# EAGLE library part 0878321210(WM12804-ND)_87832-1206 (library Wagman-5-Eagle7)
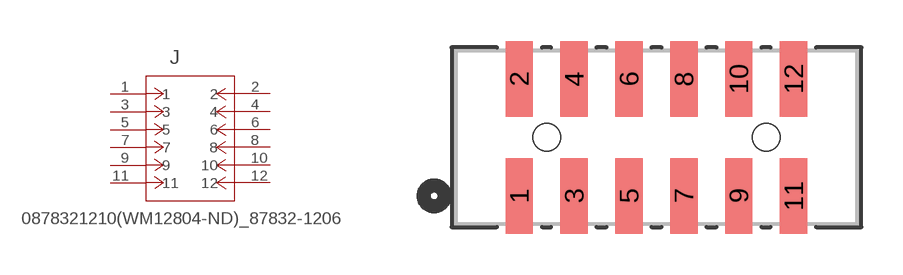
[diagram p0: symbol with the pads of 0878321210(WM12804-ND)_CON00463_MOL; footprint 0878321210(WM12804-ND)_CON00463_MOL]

Designator prefix J

## 0878321210(WM12804-ND)_87832-1206 (BUILT_BY: EMA_Don; COPYRIGHT: Copyright (C) 2016 Accelerated Designs. All rights reserved; MANUFACTURER_PART_NUMBER: 87832-1206; SOURCELIBRARY: Molex_2018-12-15; VENDOR: Molex Connector Corporation)  [0878321210(WM12804-ND)_CON00463_MOL]
1  1  pas
2  2  pas
3  3  pas
4  4  pas
5  5  pas
6  6  pas
7  7  pas
8  8  pas
9  9  pas
10  10  pas
11  11  pas
12  12  pas

## Footprint 0878321210(WM12804-ND)_CON00463_MOL (pad centres in mm)
smd 1 x 2.75: 1 -5,-2.13; 2 -5,2.13; 3 -3,-2.13; 4 -3,2.13; 5 -1,-2.13; 6 -1,2.13; 7 1,-2.13; 8 1,2.13; 9 3,-2.13; 10 3,2.13; 11 5,-2.13; 12 5,2.13
hole 1 at -4,0
hole 1 at 4,0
